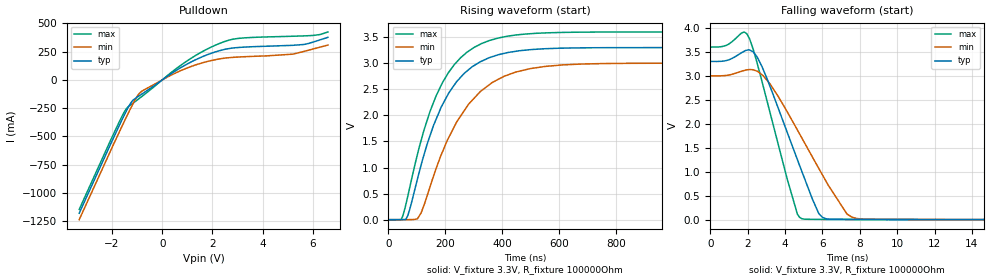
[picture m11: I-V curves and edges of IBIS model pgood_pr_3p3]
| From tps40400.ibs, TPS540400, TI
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|   pgood_pr_3p3 Model
[Model]   pgood_pr_3p3
Model_type   Open_drain
Polarity   Non-Inverting
Vmeas = 1.65
Vref = 3.3
Cref = 1pF
Rref = 100000
|   typ   min   max
C_comp   1.431pF   1.292pF   1.756pF
[Voltage Range]   3.3   3.2   3.4
[Temperature Range]   25   125   -40
[Pullup Reference]   3.3   3.2   3.4
[Pulldown Reference]   -0   -0   -0
[Power Clamp Reference]   3.3   3.2   3.4
[GND Clamp Reference]   -0   -0   -0
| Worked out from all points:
|   slope of the pulldown table from 0 to 0.495 V, typ, clamps not added: 6.57 ohm
|   falling waveform, V_fixture 3.3V, R_fixture 100000Ohm: 20-80 % time 1.9ns typ, 2.62ns min, 1.44ns max; typ from 3.3 V to 0 V
|   rising waveform, V_fixture 3.3V, R_fixture 100000Ohm: 20-80 % time 142ns typ, 169ns min, 140ns max; typ from 0 V to 3.3 V
[Pulldown]
|   Voltage   I(typ)   I(min)   I(max)
-3.3V     -1.181A    -1.238A    -1.147A
-1.518V   -316.1mA   -372.4mA   -288mA
-1.379V   -254.8mA   -308mA     -243.1mA
-1.171V   -181.7mA   -215.2mA   -207.3mA
-825mV    -127.7mA   -102mA     -149.2mA
976.8mV   138.9mA    104.5mA    166.5mA
1.769V    221mA      161.9mA    271.1mA
2.501V    271.5mA    193.4mA    341.5mA
3.194V    289.9mA    204.9mA    371.3mA
5.194V    306.5mA    228.3mA    386.9mA
5.848V    324.5mA    264.9mA    392.1mA
6.59V     377.4mA    308.9mA    424.9mA
[Ramp]
R_load = 100000
|   typ   min   max
dV/dt_r   1.97986/1.42159e-07   1.79983/1.68677e-07   2.15987/1.39735e-07
dV/dt_f   1.97986/1.90479e-09   1.79983/2.61962e-09   2.15987/1.44324e-09
[Falling Waveform]
V_fixture = 3.3V
V_fixture_min = 3V
V_fixture_max = 3.6V
R_fixture = 100000Ohm
C_fixture = 0F
|   Time   V(typ)   V(min)   V(max)
0s        3.3V       3V         3.6V
1.966ns   3.534V     3.124V     3.874V
2.291ns   3.504V     3.126V     3.565V
2.777ns   3.188V     3.02V      2.872V
4.666ns   1.251V     1.869V     114.4mV
5.808ns   127.9mV    1.07V      6.009mV
7.017ns   8.417mV    298.3mV    3.592mV
8.173ns   5.241mV    12.73mV    2.736mV
27.85ns   755.9uV    1.01mV     566uV
3us       231uV      277.1uV    214.3uV
[Rising Waveform]
V_fixture = 3.3V
V_fixture_min = 3V
V_fixture_max = 3.6V
R_fixture = 100000Ohm
C_fixture = 0F
|   Time   V(typ)   V(min)   V(max)
0s        231uV      277.1uV    214.3uV
48.89ns   8.417uV    -106.3uV   51.18mV
67.49ns   74.75mV    316.4uV    443.1mV
101.8ns   780.5mV    17.15mV    1.254V
145.6ns   1.607V     625.4mV    2.072V
210.2ns   2.415V     1.56V      2.818V
281.4ns   2.877V     2.216V     3.232V
385.4ns   3.163V     2.691V     3.484V
755.7ns   3.298V     2.994V     3.599V
3us       3.3V       3V         3.6V
